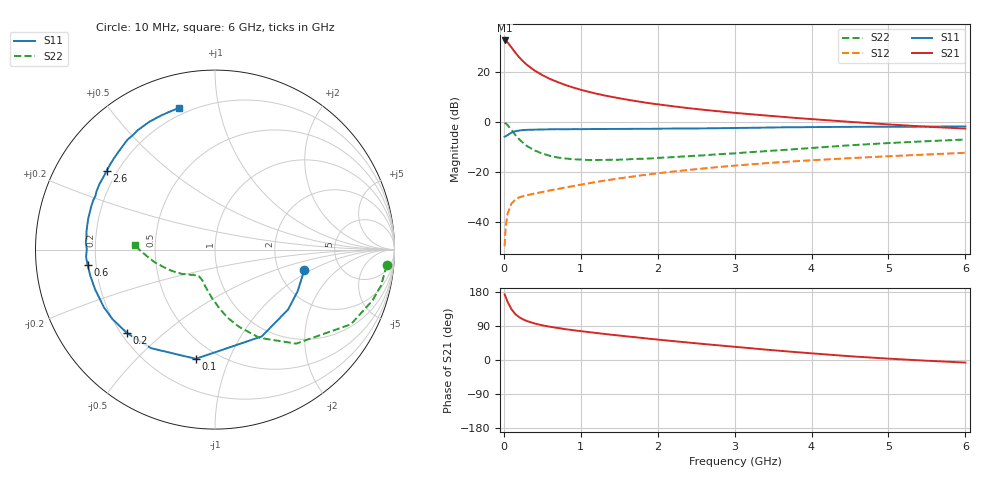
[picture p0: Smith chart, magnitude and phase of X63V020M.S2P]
! SIEMENS Small Signal Semiconductors
! BFP193W
! Si NPN RF Bipolar Junction Transistor in SOT343
! VCE = 3 V  IC = 20 mA
! Common Emitter S-Parameters:  April 1994
# GHz  S  MA  R  50
!  f  S11  S21  S12  S22
! GHz  MAG  ANG  MAG  ANG  MAG  ANG  MAG  ANG
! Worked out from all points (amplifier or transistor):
!   40 points, 10 MHz to 6 GHz, reference 50 ohm
!   highest |S21| = 32.6 dB at 10 MHz (marker M1)
!   |S21| within 3 dB of that: start of sweep to 104.5 MHz
!   unconditionally stable (mu >= 1): 949.6 MHz to 3.997 GHz
!   at 200 MHz: K = 0.35, MSG = 28.0 dB, |S12| = -30.1 dB
!   at 1.5 GHz: K = 1.11, MAG = 14.0 dB, |S12| = -22.5 dB
!   at 6 GHz: K = 0.93, MSG = 4.8 dB, |S12| = -12.3 dB
!   lowest NFmin = 1.40 dB at 450 MHz
!   S11 on the Smith chart (normalised r, x): 10 MHz: 2.78, -0.87; 100 MHz: 0.39, -0.76; 200 MHz: 0.22, -0.38; 600 MHz: 0.17, -0.06; 2.6 GHz: 0.16, +0.32; 6 GHz: 0.16, +0.77
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0.01  0.5105 -13.1  42.67 173.3  0.0033 85.7  0.9608 -5.2
0.02  0.5155 -26.8  42.28 168.4  0.0064 79.2  0.9467 -12.2
0.03  0.5266 -39.2  41.47 163.1  0.0094 76.7  0.9223 -17.9
0.05  0.5495 -61.7  38.73 152.8  0.015 66.8  0.864 -28.8
0.1  0.6179 -100.0  30.86 133.7  0.0235 52.2  0.6919 -49.2
0.15  0.6547 -123.0  24.34 121.0  0.0282 44.3  0.551 -63.2
0.2  0.6759 -136.6  19.61 112.9  0.0312 40.7  0.4516 -72.6
0.25  0.6902 -145.8  16.36 107.2  0.0329 39.0  0.3846 -79.7
0.3  0.6975 -152.5  13.88 102.8  0.0344 38.5  0.3322 -85.2
0.4  0.7041 -161.8  10.68 96.4  0.0372 38.7  0.2708 -93.5
0.5  0.7099 -168.3  8.665 91.5  0.04 40.6  0.2342 -99.9
0.6  0.7147 -173.0  7.256 87.7  0.043 42.7  0.211 -105.0
0.8  0.7143 179.9  5.496 81.4  0.0492 46.5  0.1864 -112.2
1.1  0.7232 172.1  4.036 73.7  0.0594 50.5  0.1743 -119.8
1.3  0.7256 167.6  3.42 69.0  0.067 52.1  0.1751 -123.1
1.6  0.7298 161.6  2.806 62.3  0.0785 53.4  0.1789 -127.2
2.2  0.74 150.7  2.064 49.9  0.1023 53.4  0.1985 -135.5
2.6  0.7461 144.0  1.754 42.2  0.1182 52.2  0.216 -140.9
3.2  0.7659 134.5  1.435 31.3  0.1422 49.3  0.2494 -149.2
4.5  0.8006 117.2  1.008 9.9  0.1895 41.3  0.3431 -168.1
5.5  0.8085 108.4  0.807 -1.9  0.2244 35.2  0.4135 -178.9
6  0.8149 104.2  0.739 -6.8  0.2426 32.5  0.4467 176.9
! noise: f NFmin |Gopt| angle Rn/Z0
0.45  1.4  0.3  160  0.1
0.9  1.45  0.34  172  0.11
1.8  2.2  0.56  -148  0.2
